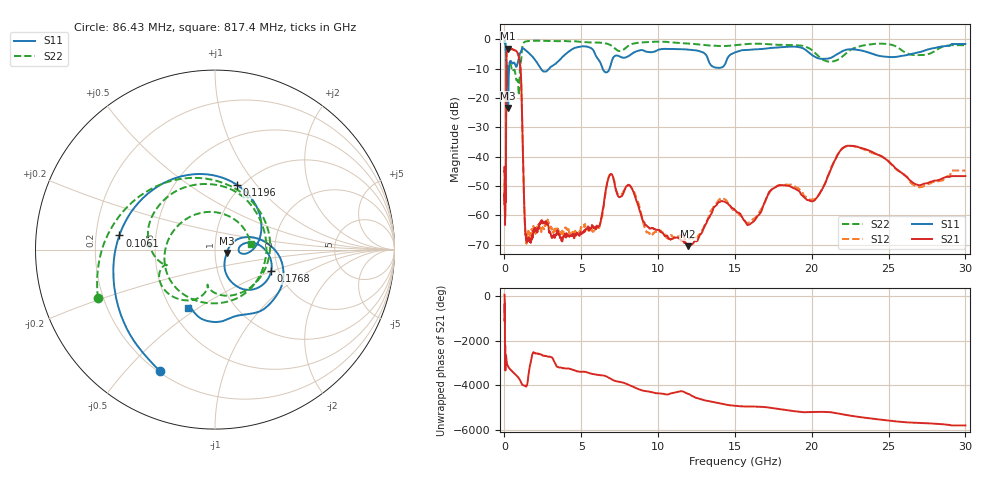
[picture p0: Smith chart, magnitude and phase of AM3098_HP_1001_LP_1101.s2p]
! Date/Time: Thu, Feb 28, 2019 8:41 AM
! Network Analyzer: Agilent Technologies E8364B Rev: A.07.50.67
! Sweep from 0.010 to 30.000 GHz, 1601 Points, Sweep Type: LOG
! Power Supply: 5.023 V, 0.002 A
# Hz S DB R 50
!freq MagS11 AngS11 MagS21 AngS21 MagS12 AngS12 MagS22 AngS22
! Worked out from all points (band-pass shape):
!   1601 points, 10 MHz to 30 GHz, reference 50 ohm
!   highest |S21| = -3.10 dB at 243.5 MHz (marker M1); lowest = -70.5 dB at 11.95 GHz (marker M2)
!   |S21| within 3 dB of the highest: 130.1 MHz to 943.5 MHz (813.3 MHz wide, 152 % of centre)
!   lowest |S11| = -23.4 dB at 239.9 MHz (marker M3), VSWR 1.15, Z = 56.9 - j2.15 ohm
!   |S11| at or under -10 dB: 192.3 MHz to 299.8 MHz (107.5 MHz wide, 43.7 % of centre); 2.371 GHz to 2.901 GHz (529.9 MHz wide, 20.1 % of centre); 6.389 GHz to 6.837 GHz (448 MHz wide, 6.77 % of centre)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
!   |S22| runs from -19.0 to -0.4 dB; largest |S21 - S12| = 0.013
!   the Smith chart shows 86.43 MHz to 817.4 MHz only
!   S11 on the Smith chart (normalised r, x): 86.43 MHz: 0.21, -0.63; 106.1 MHz: 0.30, +0.07; 119.6 MHz: 0.95, +0.80; 176.8 MHz: 1.83, -0.49; 817.4 MHz: 0.61, -0.46
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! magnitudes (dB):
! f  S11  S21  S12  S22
! 10 MHz  -0.4  -45.2  -44.7  -0.6
! 38.04 MHz  -0.5  -63.0  -60.8  -1.0
! 86.43 MHz  -2.6  -54.9  -52.5  -3.0
! 106.1 MHz  -5.4  -28.5  -28.4  -6.9
! 119.6 MHz  -8.4  -11.4  -11.4  -10.4
! 144.7 MHz  -17.3  -4.4  -4.4  -13.4
! 176.8 MHz  -9.5  -3.8  -3.7  -9.0
! 239.9 MHz  -23.4  -3.1  -3.1  -11.0
! 243.5 MHz  -23.0  -3.1  -3.1  -10.9
! 319 MHz  -8.6  -3.4  -3.3  -8.3
! 550.5 MHz  -8.1  -3.5  -3.4  -10.7
! 817.4 MHz  -8.9  -4.3  -4.2  -13.9
! 1.066 GHz  -4.3  -11.5  -11.4  -7.9
! 1.389 GHz  -3.7  -66.9  -67.8  -0.7
! 2.084 GHz  -7.6  -65.4  -64.5  -0.4
! 5.668 GHz  -3.1  -64.3  -64.7  -1.1
! 6.855 GHz  -9.7  -46.2  -46.2  -1.8
! 7.926 GHz  -6.1  -50.2  -50.2  -2.7
! 11.95 GHz  -3.5  -70.5  -67.8  -1.4
! 20.1 GHz  -5.6  -55.1  -54.6  -4.0
! 22.56 GHz  -3.4  -36.3  -36.4  -3.5
! 30 GHz  -1.6  -46.6  -44.7  -2.0
